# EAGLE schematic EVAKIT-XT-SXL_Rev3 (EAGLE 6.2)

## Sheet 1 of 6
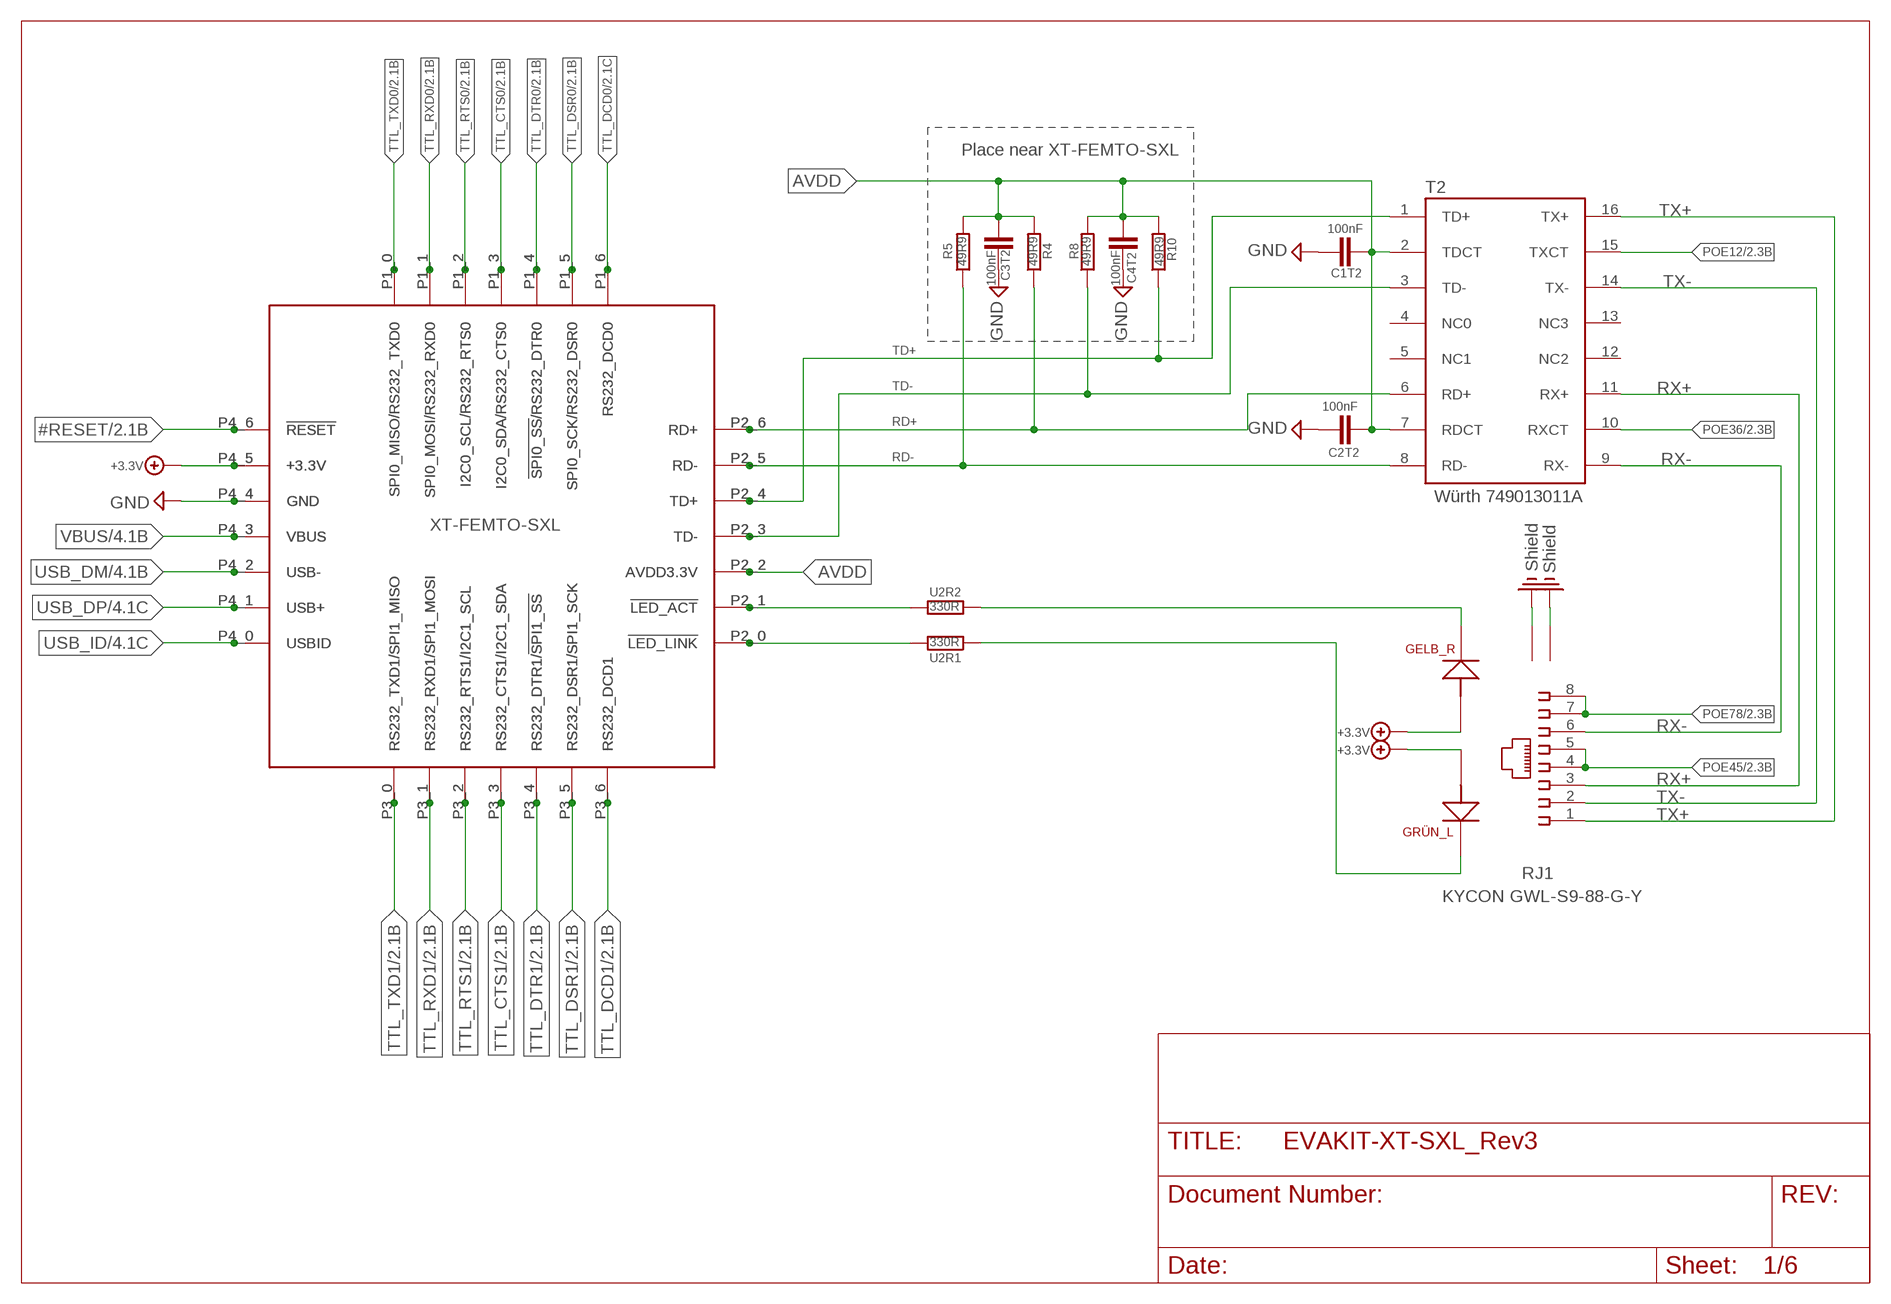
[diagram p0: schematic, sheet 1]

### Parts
C1T2  100nF  C0402AK  [AK0402]
C2T2  100nF  C0402AK  [AK0402]
C3T2  100nF  C0402AK  [AK0402]
C4T2  100nF  C0402AK  [AK0402]
M1  XT-FEMTO-SXL2  [XT-FEMTO-SXL-PAD]
R4  49R9  R0402AK  [AK0402]
R5  49R9  R0402AK  [AK0402]
R8  49R9  R0402AK  [AK0402]
R10  49R9  R0402AK  [AK0402]
RJ1  KYCON GWL-S9-88-G-Y  RJ45_ERNI_LED  [ORCAD_X_ERNI_RJ45_LED]
T2  Würth 749013011A  PULSE_H1102  [SOTRANSF]
U2R1  330R  R0402AK  [AK0402]
U2R2  330R  R0402AK  [AK0402]
XT-FEMTO-SXL  XT-FEMTO-SXL1  [XT-FEMTO-SXL-PIN]

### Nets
#RESET: M1.P4_6(!RESET) XT-FEMTO-SXL.P4_6(!RESET) ; also sheet 2,3,6
+3.3V: M1.P4_5(+3.3V) RJ1.A1 RJ1.A2 XT-FEMTO-SXL.P4_5(+3.3V) ; also sheet 2,3,4,5,6
AVDD: C1T2.1 C2T2.2 C3T2.1 C4T2.2 M1.P2_2(AVDD3.3V) R4.2 R5.2 R8.2 R10.2 T2.2(TDCT) T2.7(RDCT) XT-FEMTO-SXL.P2_2(AVDD3.3V)
GND: C1T2.2 C2T2.1 C3T2.2 C4T2.1 M1.P4_4(GND) XT-FEMTO-SXL.P4_4(GND) ; also sheet 2,3,4,5,6
N$1: M1.P2_1(!LED_ACT) U2R2.2 XT-FEMTO-SXL.P2_1(!LED_ACT)
N$2: RJ1.K2 U2R1.1
N$4: RJ1.K1 U2R2.1
N$6: M1.P2_0(!LED_LINK) U2R1.2 XT-FEMTO-SXL.P2_0(!LED_LINK)
PE: RJ1.9 RJ1.10 ; supply symbol labelled Shield ; also sheet 2,3,4,5
POE12: T2.15(TXCT) ; also sheet 2,3,6
POE36: T2.10(RXCT) ; also sheet 2,3,6
POE45: RJ1.4 RJ1.5 ; also sheet 2,3,6
POE78: RJ1.7 RJ1.8 ; also sheet 2,3,6
RD+: M1.P2_6(RD+) R4.1 T2.6(RD+) XT-FEMTO-SXL.P2_6(RD+)
RD-: M1.P2_5(RD-) R5.1 T2.8(RD-) XT-FEMTO-SXL.P2_5(RD-)
RX+: RJ1.3 T2.11(RX+)
RX-: RJ1.6 T2.9(RX-)
TD+: M1.P2_4(TD+) R10.1 T2.1(TD+) XT-FEMTO-SXL.P2_4(TD+)
TD-: M1.P2_3(TD-) R8.1 T2.3(TD-) XT-FEMTO-SXL.P2_3(TD-)
TTL_CTS0: M1.P1_3(I2C0_SDA/RS232_CTS0) XT-FEMTO-SXL.P1_3(I2C0_SDA/RS232_CTS0) ; also sheet 2,3,6
TTL_CTS1: M1.P3_3(RS232_CTS1/I2C1_SDA) XT-FEMTO-SXL.P3_3(RS232_CTS1/I2C1_SDA) ; also sheet 2,3,6
TTL_DCD0: M1.P1_6(RS232_DCD0) XT-FEMTO-SXL.P1_6(RS232_DCD0) ; also sheet 2,3,6
TTL_DCD1: M1.P3_6(RS232_DCD1) XT-FEMTO-SXL.P3_6(RS232_DCD1) ; also sheet 2,3,6
TTL_DSR0: M1.P1_5(SPI0_SCK/RS232_DSR0) XT-FEMTO-SXL.P1_5(SPI0_SCK/RS232_DSR0) ; also sheet 2,3,6
TTL_DSR1: M1.P3_5(RS232_DSR1/SPI1_SCK) XT-FEMTO-SXL.P3_5(RS232_DSR1/SPI1_SCK) ; also sheet 2,3,6
TTL_DTR0: M1.P1_4(!SPI0_SS!/RS232_DTR0) XT-FEMTO-SXL.P1_4(!SPI0_SS!/RS232_DTR0) ; also sheet 2,3,6
TTL_DTR1: M1.P3_4(RS232_DTR1/!SPI1_SS!) XT-FEMTO-SXL.P3_4(RS232_DTR1/!SPI1_SS!) ; also sheet 2,3,6
TTL_RTS0: M1.P1_2(I2C0_SCL/RS232_RTS0) XT-FEMTO-SXL.P1_2(I2C0_SCL/RS232_RTS0) ; also sheet 2,3,6
TTL_RTS1: M1.P3_2(RS232_RTS1/I2C1_SCL) XT-FEMTO-SXL.P3_2(RS232_RTS1/I2C1_SCL) ; also sheet 2,3,6
TTL_RXD0: M1.P1_1(SPI0_MOSI/RS232_RXD0) XT-FEMTO-SXL.P1_1(SPI0_MOSI/RS232_RXD0) ; also sheet 2,3,6
TTL_RXD1: M1.P3_1(RS232_RXD1/SPI1_MOSI) XT-FEMTO-SXL.P3_1(RS232_RXD1/SPI1_MOSI) ; also sheet 2,3,6
TTL_TXD0: M1.P1_0(SPI0_MISO/RS232_TXD0) XT-FEMTO-SXL.P1_0(SPI0_MISO/RS232_TXD0) ; also sheet 2,3,6
TTL_TXD1: M1.P3_0(RS232_TXD1/SPI1_MISO) XT-FEMTO-SXL.P3_0(RS232_TXD1/SPI1_MISO) ; also sheet 2,3,6
TX+: RJ1.1 T2.16(TX+)
TX-: RJ1.2 T2.14(TX-)
USB_DM: M1.P4_2(USB-) XT-FEMTO-SXL.P4_2(USB-) ; also sheet 4
USB_DP: M1.P4_1(USB+) XT-FEMTO-SXL.P4_1(USB+) ; also sheet 4
USB_ID: M1.P4_0(USBID) XT-FEMTO-SXL.P4_0(USBID) ; also sheet 4
VBUS: M1.P4_3(VBUS) XT-FEMTO-SXL.P4_3(VBUS) ; also sheet 4
Unconnected: T2.4(NC0) T2.5(NC1) T2.12(NC2) T2.13(NC3)

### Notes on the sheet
- Place near XT-FEMTO-SXL

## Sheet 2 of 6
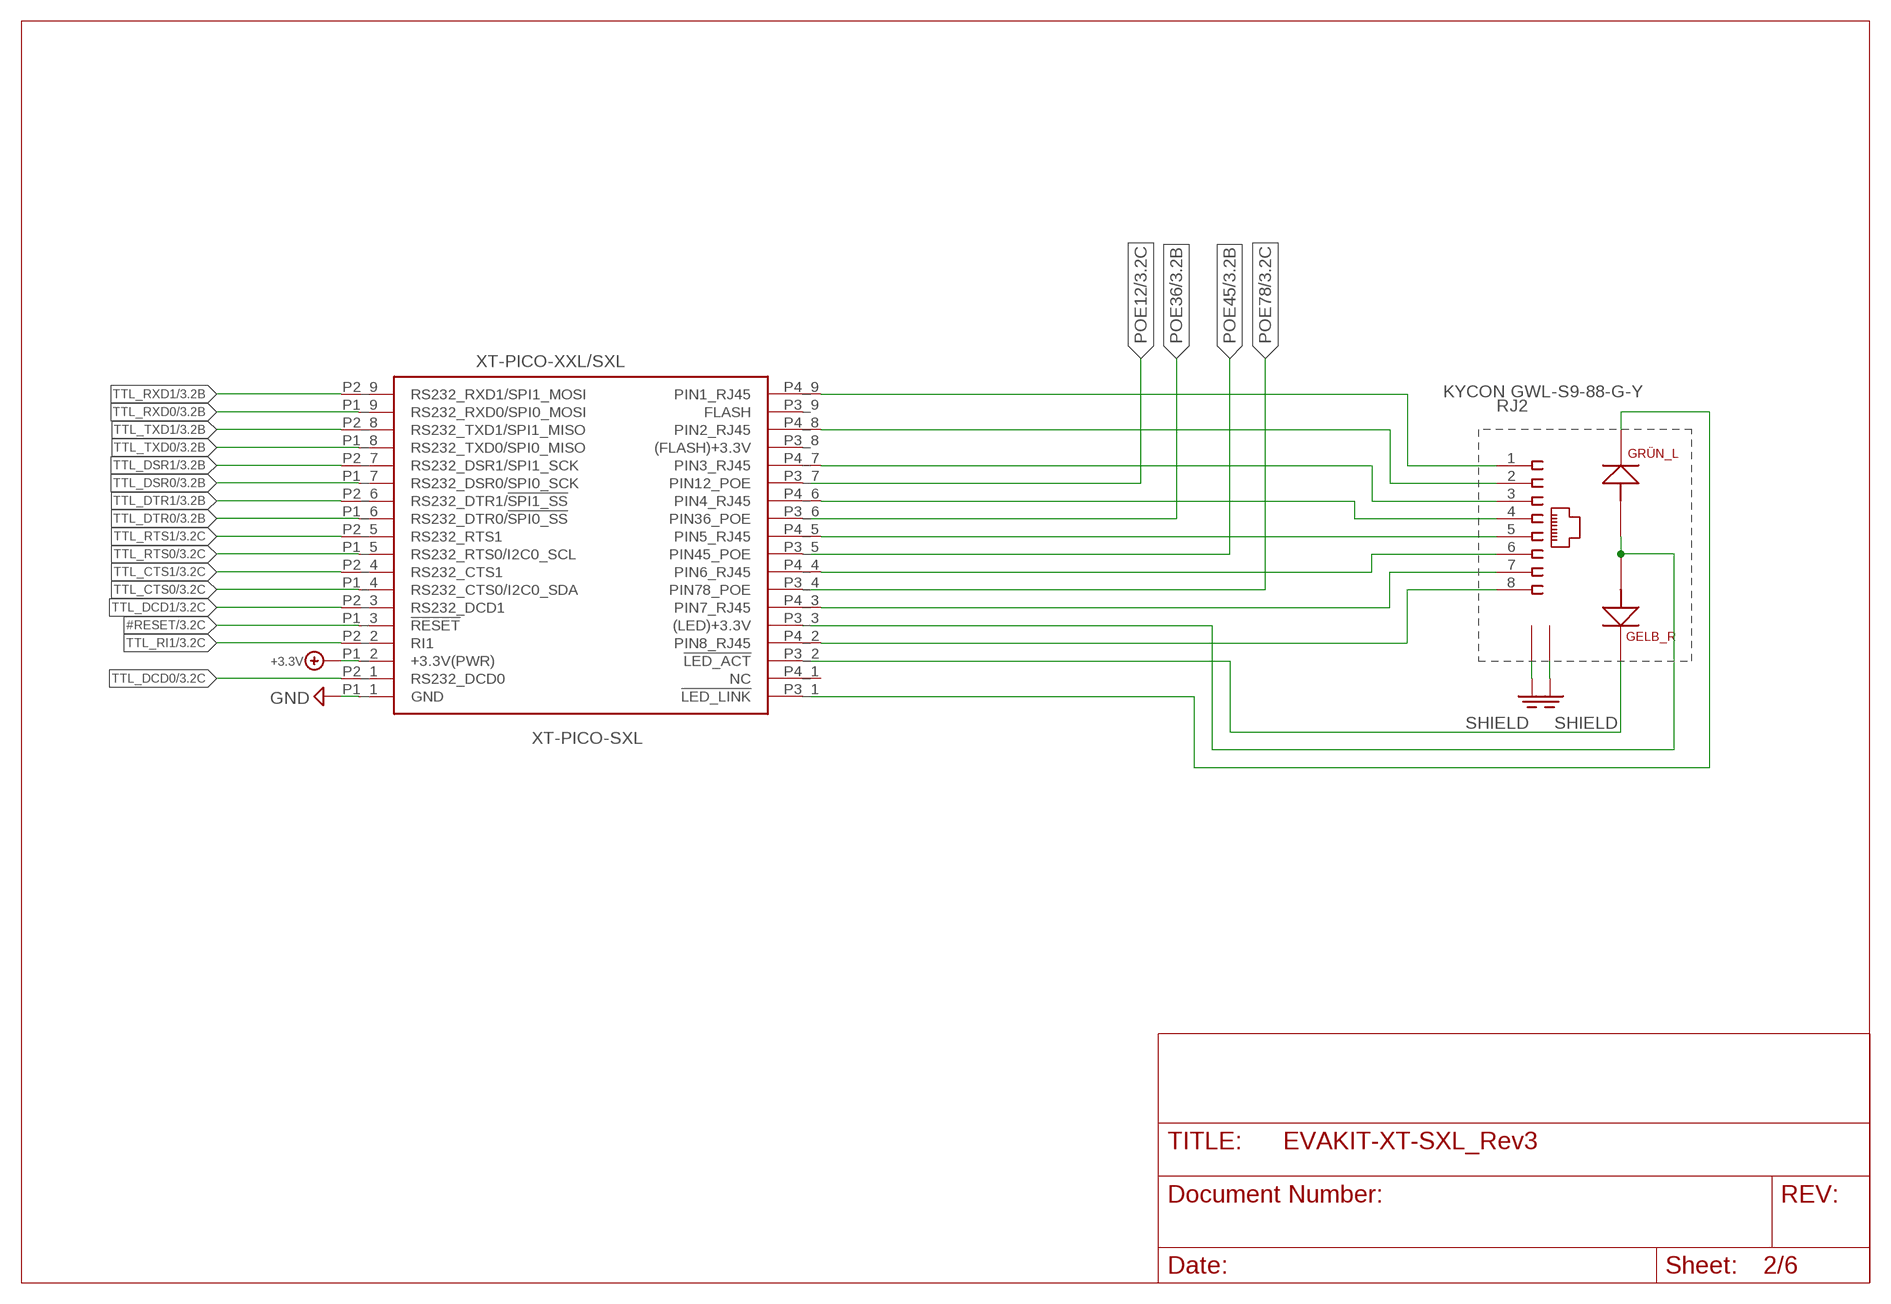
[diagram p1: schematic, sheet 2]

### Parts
RJ2  KYCON GWL-S9-88-G-Y  RJ45_ERNI_LED  [ORCAD_X_ERNI_RJ45_LED]
XT-PICO-SXL  XT-PICO-XXL/SXL  [XT-PICO-XXL/SXL]

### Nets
#RESET: XT-PICO-SXL.P1_3(!RESET) ; also sheet 1,3,6
+3.3V: XT-PICO-SXL.P1_2(+3.3V(PWR)) ; also sheet 1,3,4,5,6
GND: XT-PICO-SXL.P1_1(GND) ; also sheet 1,3,4,5,6
N$23: RJ2.1 XT-PICO-SXL.P4_9(PIN1_RJ45)
N$24: RJ2.2 XT-PICO-SXL.P4_8(PIN2_RJ45)
N$25: RJ2.3 XT-PICO-SXL.P4_7(PIN3_RJ45)
N$26: RJ2.6 XT-PICO-SXL.P4_4(PIN6_RJ45)
N$27: RJ2.K1 XT-PICO-SXL.P3_2(!LED_ACT)
N$28: RJ2.K2 XT-PICO-SXL.P3_1(!LED_LINK)
N$29: RJ2.A1 RJ2.A2 XT-PICO-SXL.P3_3((LED)+3.3V)
N$34: RJ2.4 XT-PICO-SXL.P4_6(PIN4_RJ45)
N$35: RJ2.5 XT-PICO-SXL.P4_5(PIN5_RJ45)
N$36: RJ2.7 XT-PICO-SXL.P4_3(PIN7_RJ45)
N$39: RJ2.8 XT-PICO-SXL.P4_2(PIN8_RJ45)
PE: RJ2.9 RJ2.10 ; supply symbol labelled SHIELD ; also sheet 1,3,4,5
POE12: XT-PICO-SXL.P3_7(PIN12_POE) ; also sheet 1,3,6
POE36: XT-PICO-SXL.P3_6(PIN36_POE) ; also sheet 1,3,6
POE45: XT-PICO-SXL.P3_5(PIN45_POE) ; also sheet 1,3,6
POE78: XT-PICO-SXL.P3_4(PIN78_POE) ; also sheet 1,3,6
TTL_CTS0: XT-PICO-SXL.P1_4(RS232_CTS0/I2C0_SDA) ; also sheet 1,3,6
TTL_CTS1: XT-PICO-SXL.P2_4(RS232_CTS1) ; also sheet 1,3,6
TTL_DCD0: XT-PICO-SXL.P2_1(RS232_DCD0) ; also sheet 1,3,6
TTL_DCD1: XT-PICO-SXL.P2_3(RS232_DCD1) ; also sheet 1,3,6
TTL_DSR0: XT-PICO-SXL.P1_7(RS232_DSR0/SPI0_SCK) ; also sheet 1,3,6
TTL_DSR1: XT-PICO-SXL.P2_7(RS232_DSR1/SPI1_SCK) ; also sheet 1,3,6
TTL_DTR0: XT-PICO-SXL.P1_6(RS232_DTR0/!SPI0_SS!) ; also sheet 1,3,6
TTL_DTR1: XT-PICO-SXL.P2_6(RS232_DTR1/!SPI1_SS!) ; also sheet 1,3,6
TTL_RI1: XT-PICO-SXL.P2_2(RI1) ; also sheet 3,6
TTL_RTS0: XT-PICO-SXL.P1_5(RS232_RTS0/I2C0_SCL) ; also sheet 1,3,6
TTL_RTS1: XT-PICO-SXL.P2_5(RS232_RTS1) ; also sheet 1,3,6
TTL_RXD0: XT-PICO-SXL.P1_9(RS232_RXD0/SPI0_MOSI) ; also sheet 1,3,6
TTL_RXD1: XT-PICO-SXL.P2_9(RS232_RXD1/SPI1_MOSI) ; also sheet 1,3,6
TTL_TXD0: XT-PICO-SXL.P1_8(RS232_TXD0/SPI0_MISO) ; also sheet 1,3,6
TTL_TXD1: XT-PICO-SXL.P2_8(RS232_TXD1/SPI1_MISO) ; also sheet 1,3,6
Unconnected: XT-PICO-SXL.P3_8((FLASH)+3.3V) XT-PICO-SXL.P3_9(FLASH) XT-PICO-SXL.P4_1(NC)

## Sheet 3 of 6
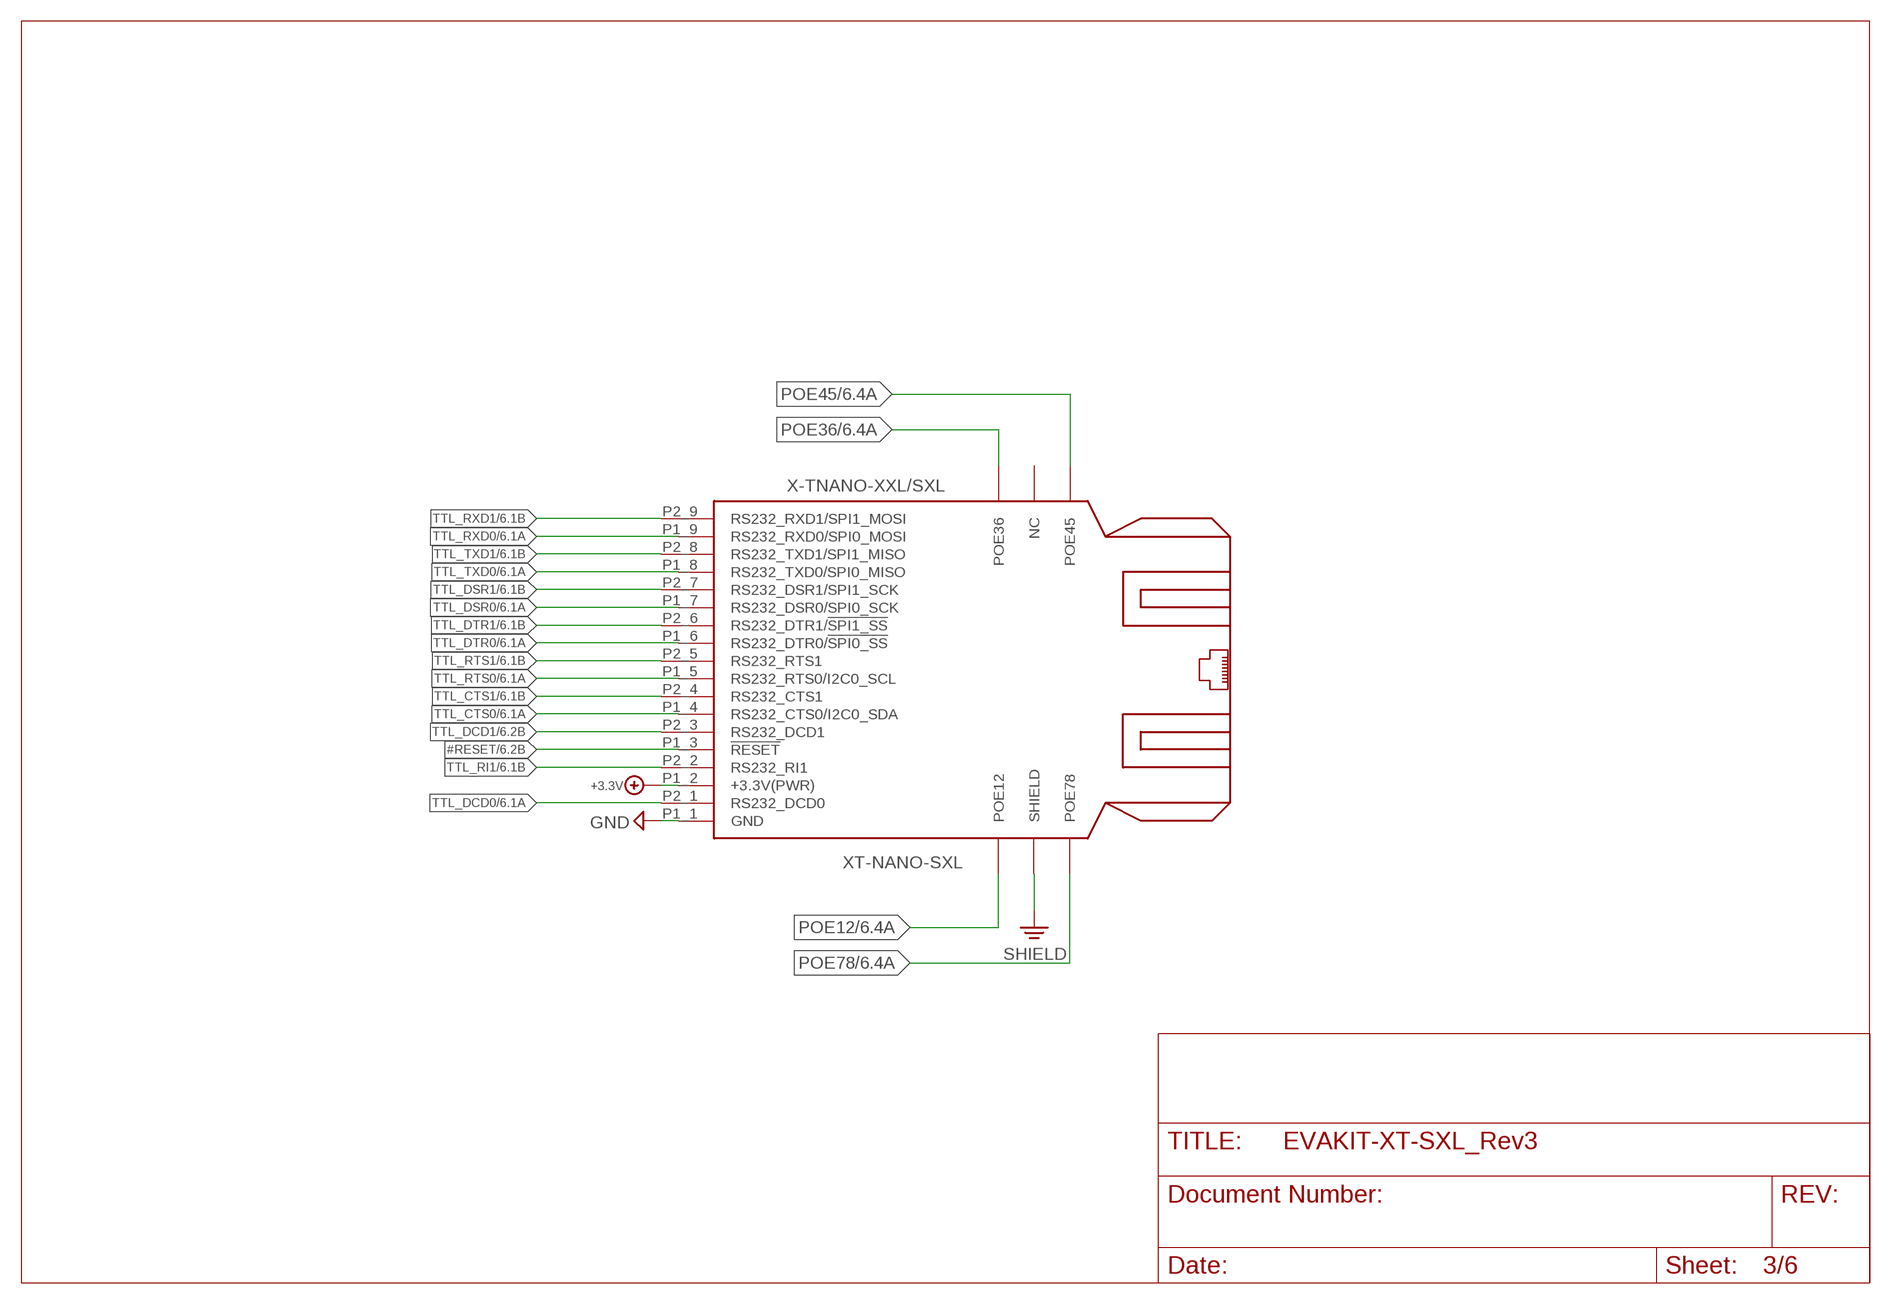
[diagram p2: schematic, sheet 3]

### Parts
XT-NANO-SXL  X-TNANO-XXL/SXL  [XT-NANO-XXL/SXL]

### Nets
#RESET: XT-NANO-SXL.P1_3(!RESET) ; also sheet 1,2,6
+3.3V: XT-NANO-SXL.P1_2(+3.3V(PWR)) ; also sheet 1,2,4,5,6
GND: XT-NANO-SXL.P1_1(GND) ; also sheet 1,2,4,5,6
PE: XT-NANO-SXL.SHIELD ; supply symbol labelled SHIELD ; also sheet 1,2,4,5
POE12: XT-NANO-SXL.POE12 ; also sheet 1,2,6
POE36: XT-NANO-SXL.POE36 ; also sheet 1,2,6
POE45: XT-NANO-SXL.POE45 ; also sheet 1,2,6
POE78: XT-NANO-SXL.POE78 ; also sheet 1,2,6
TTL_CTS0: XT-NANO-SXL.P1_4(RS232_CTS0/I2C0_SDA) ; also sheet 1,2,6
TTL_CTS1: XT-NANO-SXL.P2_4(RS232_CTS1) ; also sheet 1,2,6
TTL_DCD0: XT-NANO-SXL.P2_1(RS232_DCD0) ; also sheet 1,2,6
TTL_DCD1: XT-NANO-SXL.P2_3(RS232_DCD1) ; also sheet 1,2,6
TTL_DSR0: XT-NANO-SXL.P1_7(RS232_DSR0/SPI0_SCK) ; also sheet 1,2,6
TTL_DSR1: XT-NANO-SXL.P2_7(RS232_DSR1/SPI1_SCK) ; also sheet 1,2,6
TTL_DTR0: XT-NANO-SXL.P1_6(RS232_DTR0/!SPI0_SS!) ; also sheet 1,2,6
TTL_DTR1: XT-NANO-SXL.P2_6(RS232_DTR1/!SPI1_SS!) ; also sheet 1,2,6
TTL_RI1: XT-NANO-SXL.P2_2(RS232_RI1) ; also sheet 2,6
TTL_RTS0: XT-NANO-SXL.P1_5(RS232_RTS0/I2C0_SCL) ; also sheet 1,2,6
TTL_RTS1: XT-NANO-SXL.P2_5(RS232_RTS1) ; also sheet 1,2,6
TTL_RXD0: XT-NANO-SXL.P1_9(RS232_RXD0/SPI0_MOSI) ; also sheet 1,2,6
TTL_RXD1: XT-NANO-SXL.P2_9(RS232_RXD1/SPI1_MOSI) ; also sheet 1,2,6
TTL_TXD0: XT-NANO-SXL.P1_8(RS232_TXD0/SPI0_MISO) ; also sheet 1,2,6
TTL_TXD1: XT-NANO-SXL.P2_8(RS232_TXD1/SPI1_MISO) ; also sheet 1,2,6
Unconnected: XT-NANO-SXL.FLASH(NC)

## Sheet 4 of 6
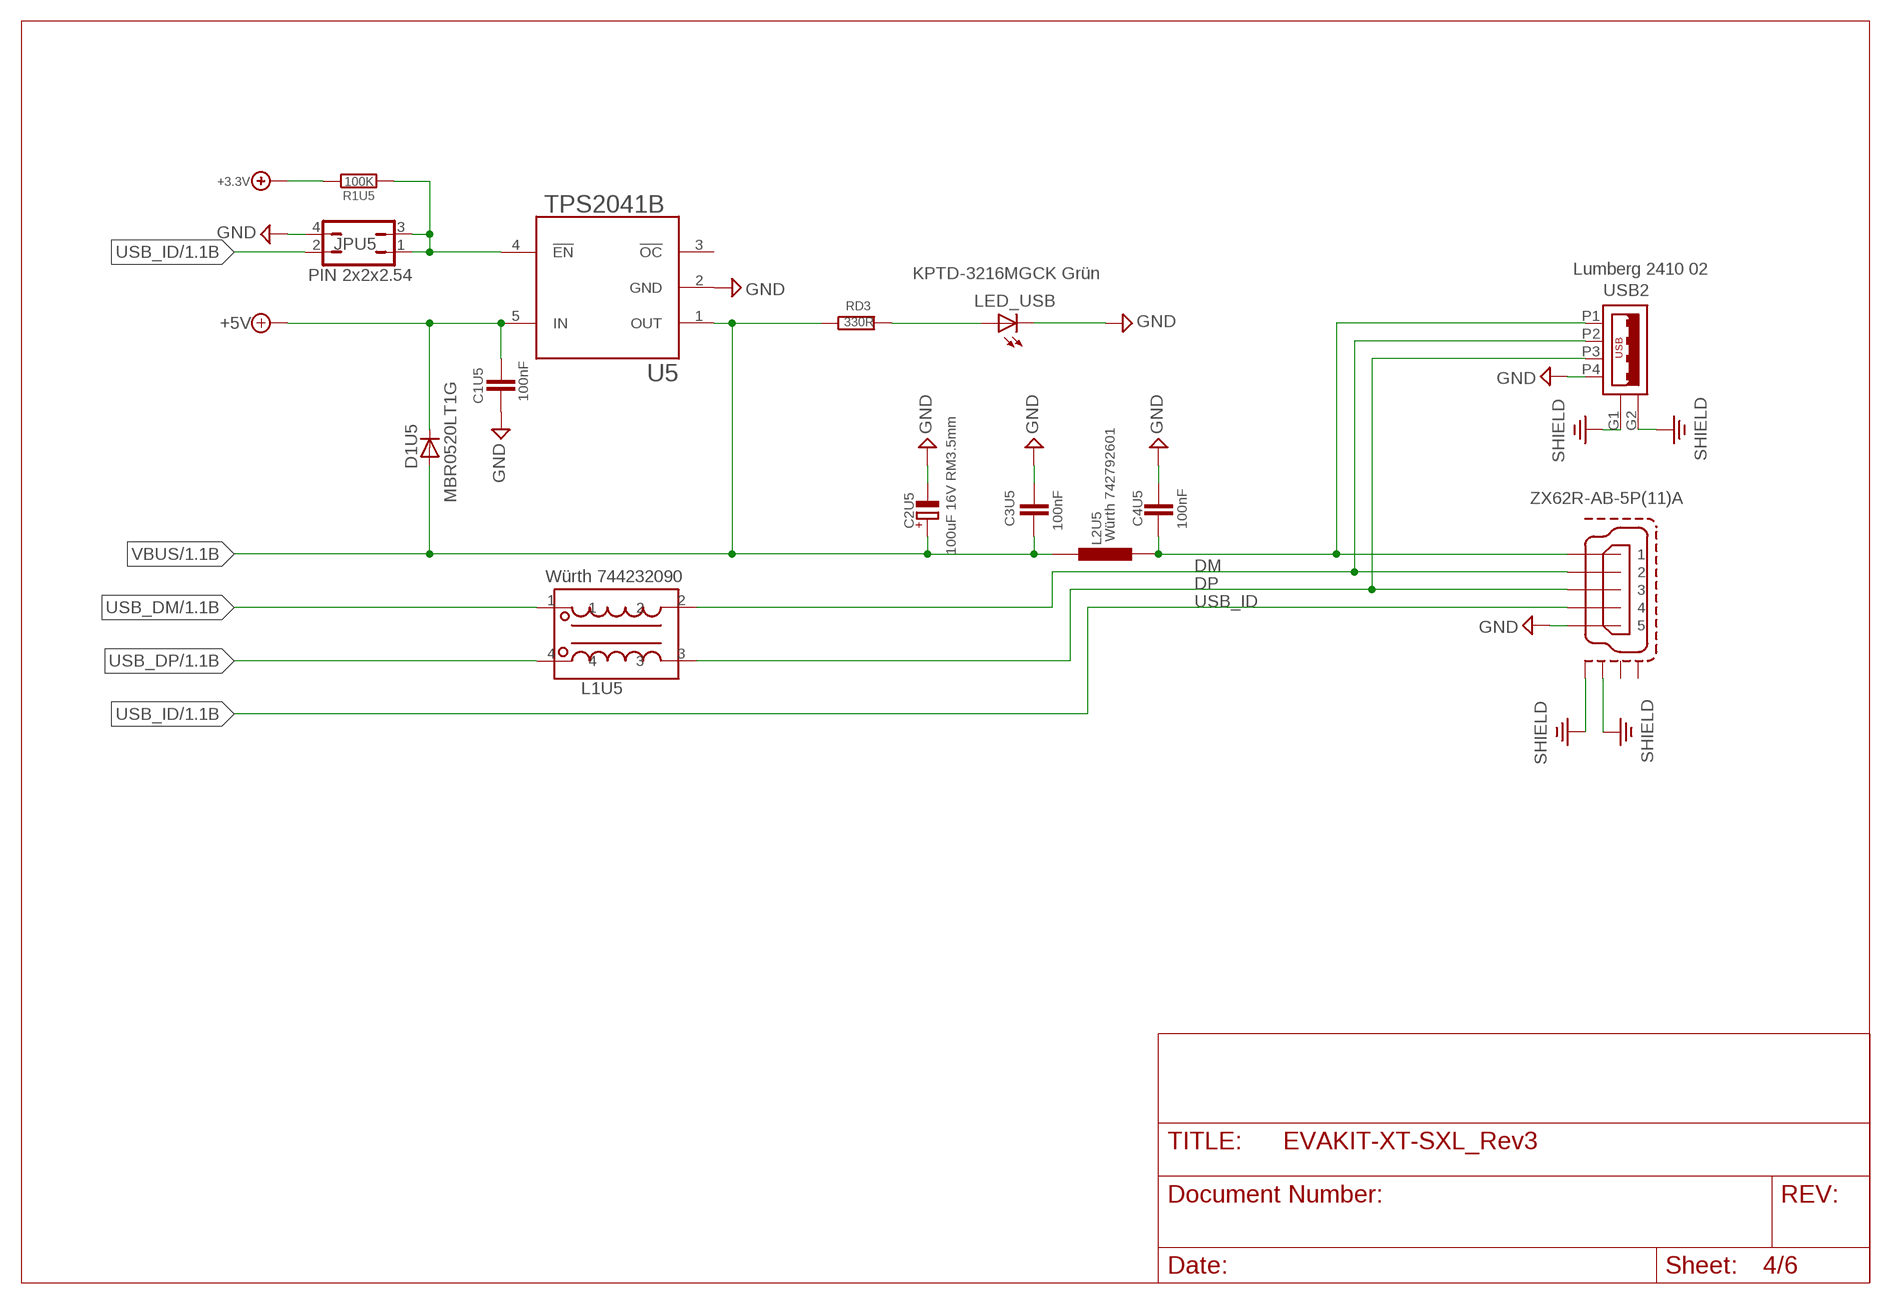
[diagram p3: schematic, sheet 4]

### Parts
C1U5  100nF  C0402AK  [AK0402]
C2U5  100uF 16V RM3.5mm  CPOL-EU153CLV-0605  [153CLV-0605]
C3U5  100nF  C0402AK  [AK0402]
C4U5  100nF  C0402AK  [AK0402]
D1U5  MBR0520LT1G  MBR0520LT  [SOD123]
JPU5  PIN 2x2x2.54  JP2Q  [JP2Q]
L1U5  Würth 744232090  WE-CNSW  [2L1206]
L2U5  Würth 742792601  CHIP-L-0603  [SMD-0603]
LED_USB  KPTD-3216MGCK Grün  LEDSMT1206  [1206]
R1U5  100K  R0402AK  [AK0402]
RD3  330R  R0402AK  [AK0402]
U5  TPS2041B  [SOT23-5]
USB1  ZX62R-AB-5P(11)A  [ZX62R-AB-5P(11)]
USB2  Lumberg 2410 02  USB_A_1  [USB_A_1]

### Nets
+3.3V: R1U5.1 ; also sheet 1,2,3,5,6
+5V: C1U5.1 D1U5.C U5.5(IN) ; also sheet 6
DM: L1U5.2 USB1.2 USB2.P2
DP: L1U5.3 USB1.3 USB2.P3
GND: C1U5.2 C2U5.- C3U5.1 C4U5.1 JPU5.4 LED_USB.C U5.2(GND) USB1.5 USB2.P4 ; also sheet 1,2,3,5,6
N$15: C4U5.2 L2U5.2 USB1.1 USB2.P1
N$16: JPU5.1 JPU5.3 R1U5.2 U5.4(!EN)
N$22: LED_USB.A RD3.2
PE: USB1.M1(S1) USB1.M2(S2) USB2.G1 USB2.G2 ; supply symbol labelled SHIELD ; also sheet 1,2,3,5
USB_DM: L1U5.1 ; also sheet 1
USB_DP: L1U5.4 ; also sheet 1
USB_ID: JPU5.2 USB1.4 ; also sheet 1
VBUS: C2U5.+ C3U5.2 D1U5.A L2U5.1 RD3.1 U5.1(OUT) ; also sheet 1
Unconnected: U5.3(!OC) USB1.M3(S3) USB1.M4(S4)

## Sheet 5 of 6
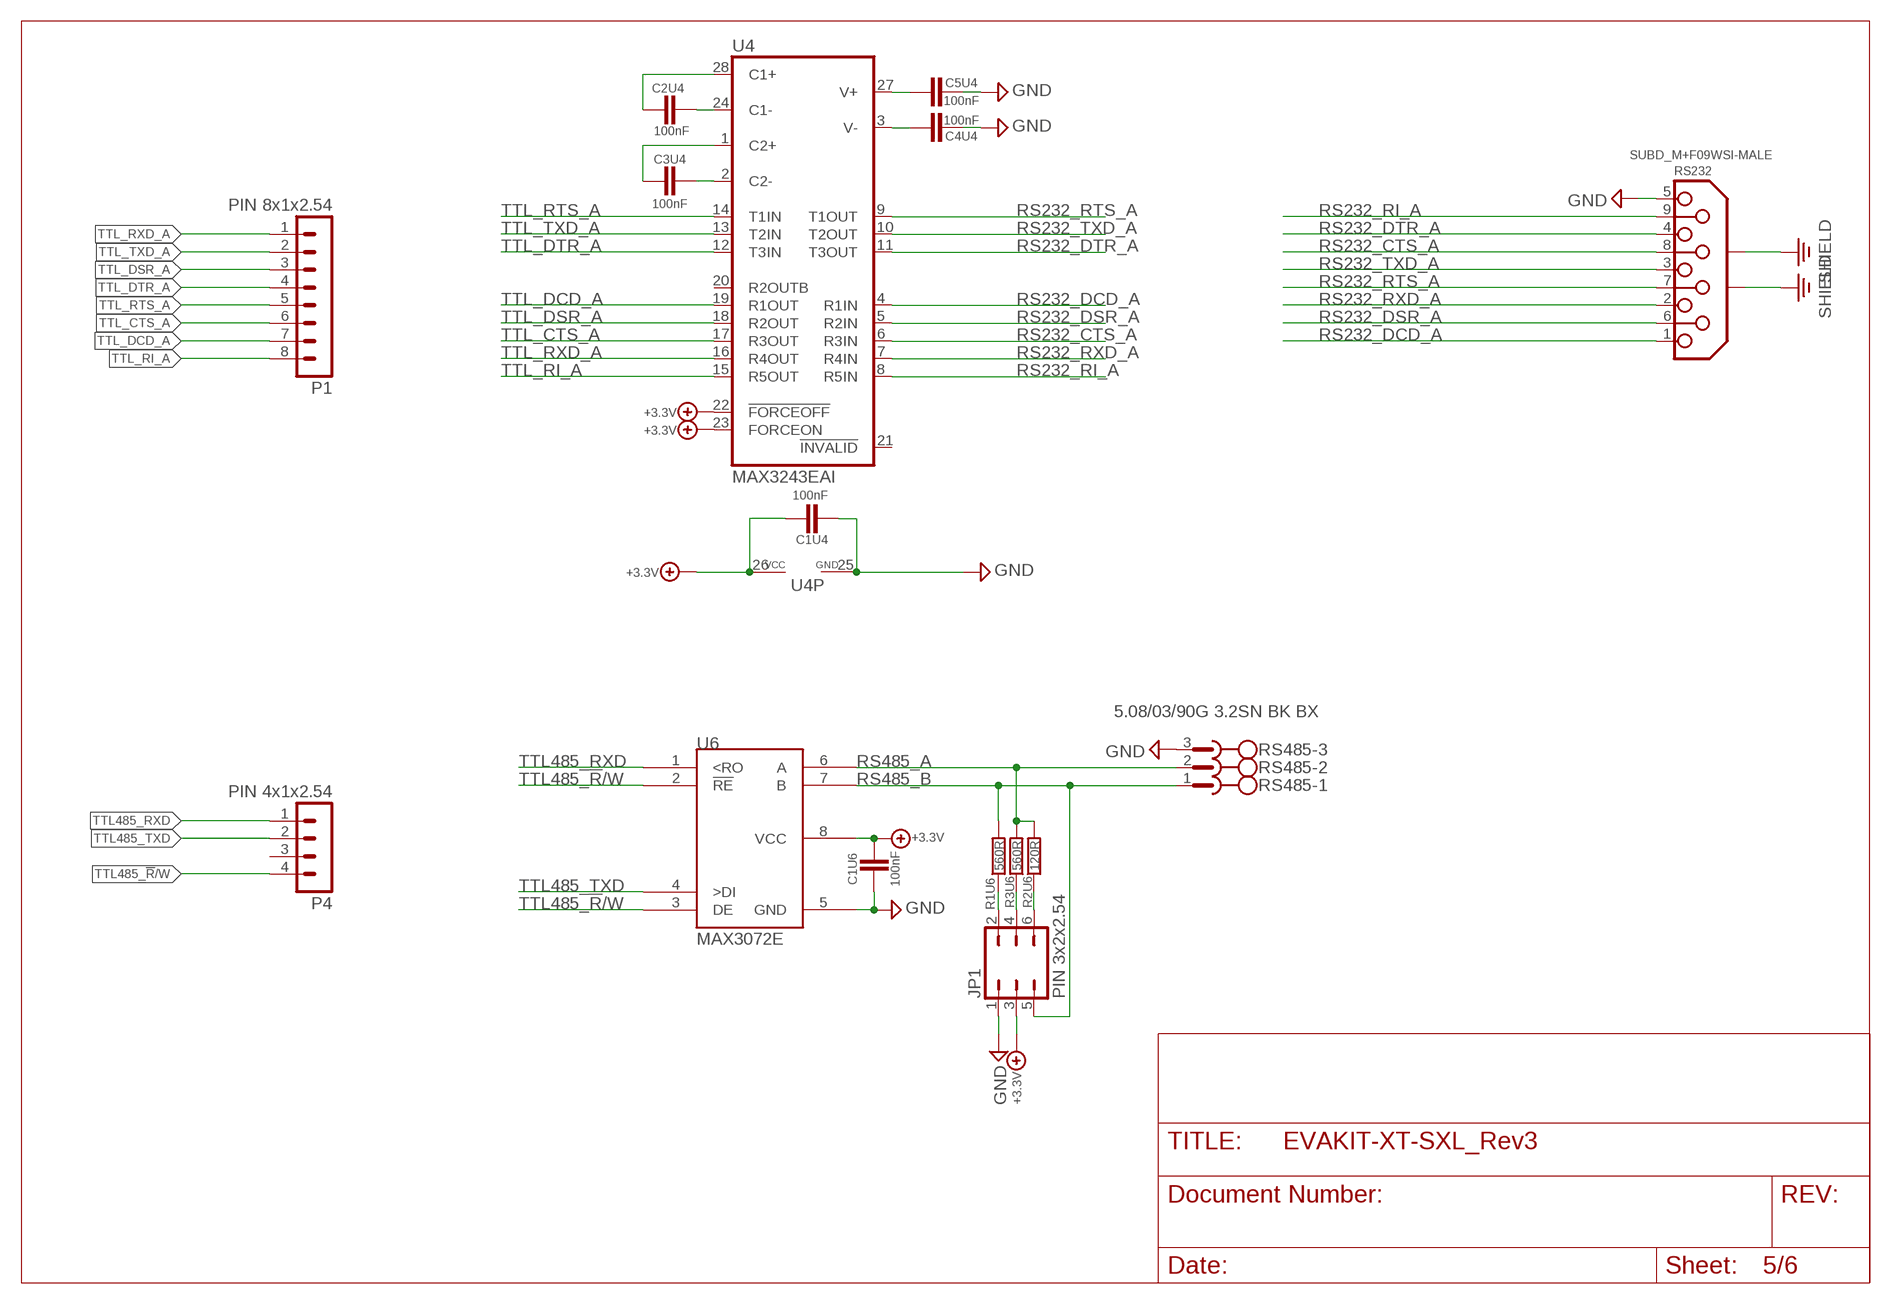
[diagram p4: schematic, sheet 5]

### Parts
C1U4  100nF  C0402AK  [AK0402]
C1U6  100nF  C0402AK  [AK0402]
C2U4  100nF  C0402AK  [AK0402]
C3U4  100nF  C0402AK  [AK0402]
C4U4  100nF  C0402AK  [AK0402]
C5U4  100nF  C0402AK  [AK0402]
JP1  PIN 3x2x2.54  JP3Q  [JP3Q]
P1  PIN 8x1x2.54  MA08-1  [MA08-1]
P4  PIN 4x1x2.54  MA04-1  [MA04-1]
R1U6  560R  R0402AK  [AK0402]
R2U6  120R  R0402AK  [AK0402]
R3U6  560R  R0402AK  [AK0402]
RS232  SUBD_M+F09WSI-MALE  [SUBD-M09HP-WSI]
RS485  5.08/03/90G 3.2SN BK BX  MSTBA3  [MSTBA3]
U4  MAX3243EAI  [SSOP28]
U6  MAX3072E  MAX3072E_SO8  [SO-8]

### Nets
+3.3V: C1U4.1 C1U6.2 JP1.3 U4.22(!FORCEOFF) U4.23(FORCEON) U4.26(VCC) U6.8(VCC) ; also sheet 1,2,3,4,6
GND: C1U4.2 C1U6.1 C4U4.2 C5U4.2 JP1.1 RS232.5 RS485.3 U4.25(GND) U6.5(GND) ; also sheet 1,2,3,4,6
N$3: C2U4.2 U4.28(C1+)
N$8: C3U4.2 U4.1(C2+)
N$10: C3U4.1 U4.2(C2-)
N$12: C2U4.1 U4.24(C1-)
N$13: C5U4.1 U4.27(V+)
N$14: C4U4.1 U4.3(V-)
N$17: JP1.2 R1U6.1
N$18: JP1.6 R2U6.1
N$19: JP1.4 R3U6.1
PE: RS232.G1 RS232.G2 ; supply symbol labelled SHIELD ; also sheet 1,2,3,4
RS232_CTS_A: RS232.8 U4.6(R3IN)
RS232_DCD_A: RS232.1 U4.4(R1IN)
RS232_DSR_A: RS232.6 U4.5(R2IN)
RS232_DTR_A: RS232.4 U4.11(T3OUT)
RS232_RI_A: RS232.9 U4.8(R5IN)
RS232_RTS_A: RS232.7 U4.9(T1OUT)
RS232_RXD_A: RS232.2 U4.7(R4IN)
RS232_TXD_A: RS232.3 U4.10(T2OUT)
RS485_A: R2U6.2 R3U6.2 RS485.2 U6.6(A)
RS485_B: JP1.5 R1U6.2 RS485.1 U6.7(B)
TTL485_!R!/W: P4.4 U6.2(!RE) U6.3(DE)
TTL485_RXD: P4.1 U6.1(<RO)
TTL485_TXD: P4.2 U6.4(>DI)
TTL_CTS_A: P1.6 U4.17(R3OUT)
TTL_DCD_A: P1.7 U4.19(R1OUT)
TTL_DSR_A: P1.3 U4.18(R2OUT)
TTL_DTR_A: P1.4 U4.12(T3IN)
TTL_RI_A: P1.8 U4.15(R5OUT)
TTL_RTS_A: P1.5 U4.14(T1IN)
TTL_RXD_A: P1.1 U4.16(R4OUT)
TTL_TXD_A: P1.2 U4.13(T2IN)
Unconnected: P4.3 U4.20(R2OUTB) U4.21(!INVALID)

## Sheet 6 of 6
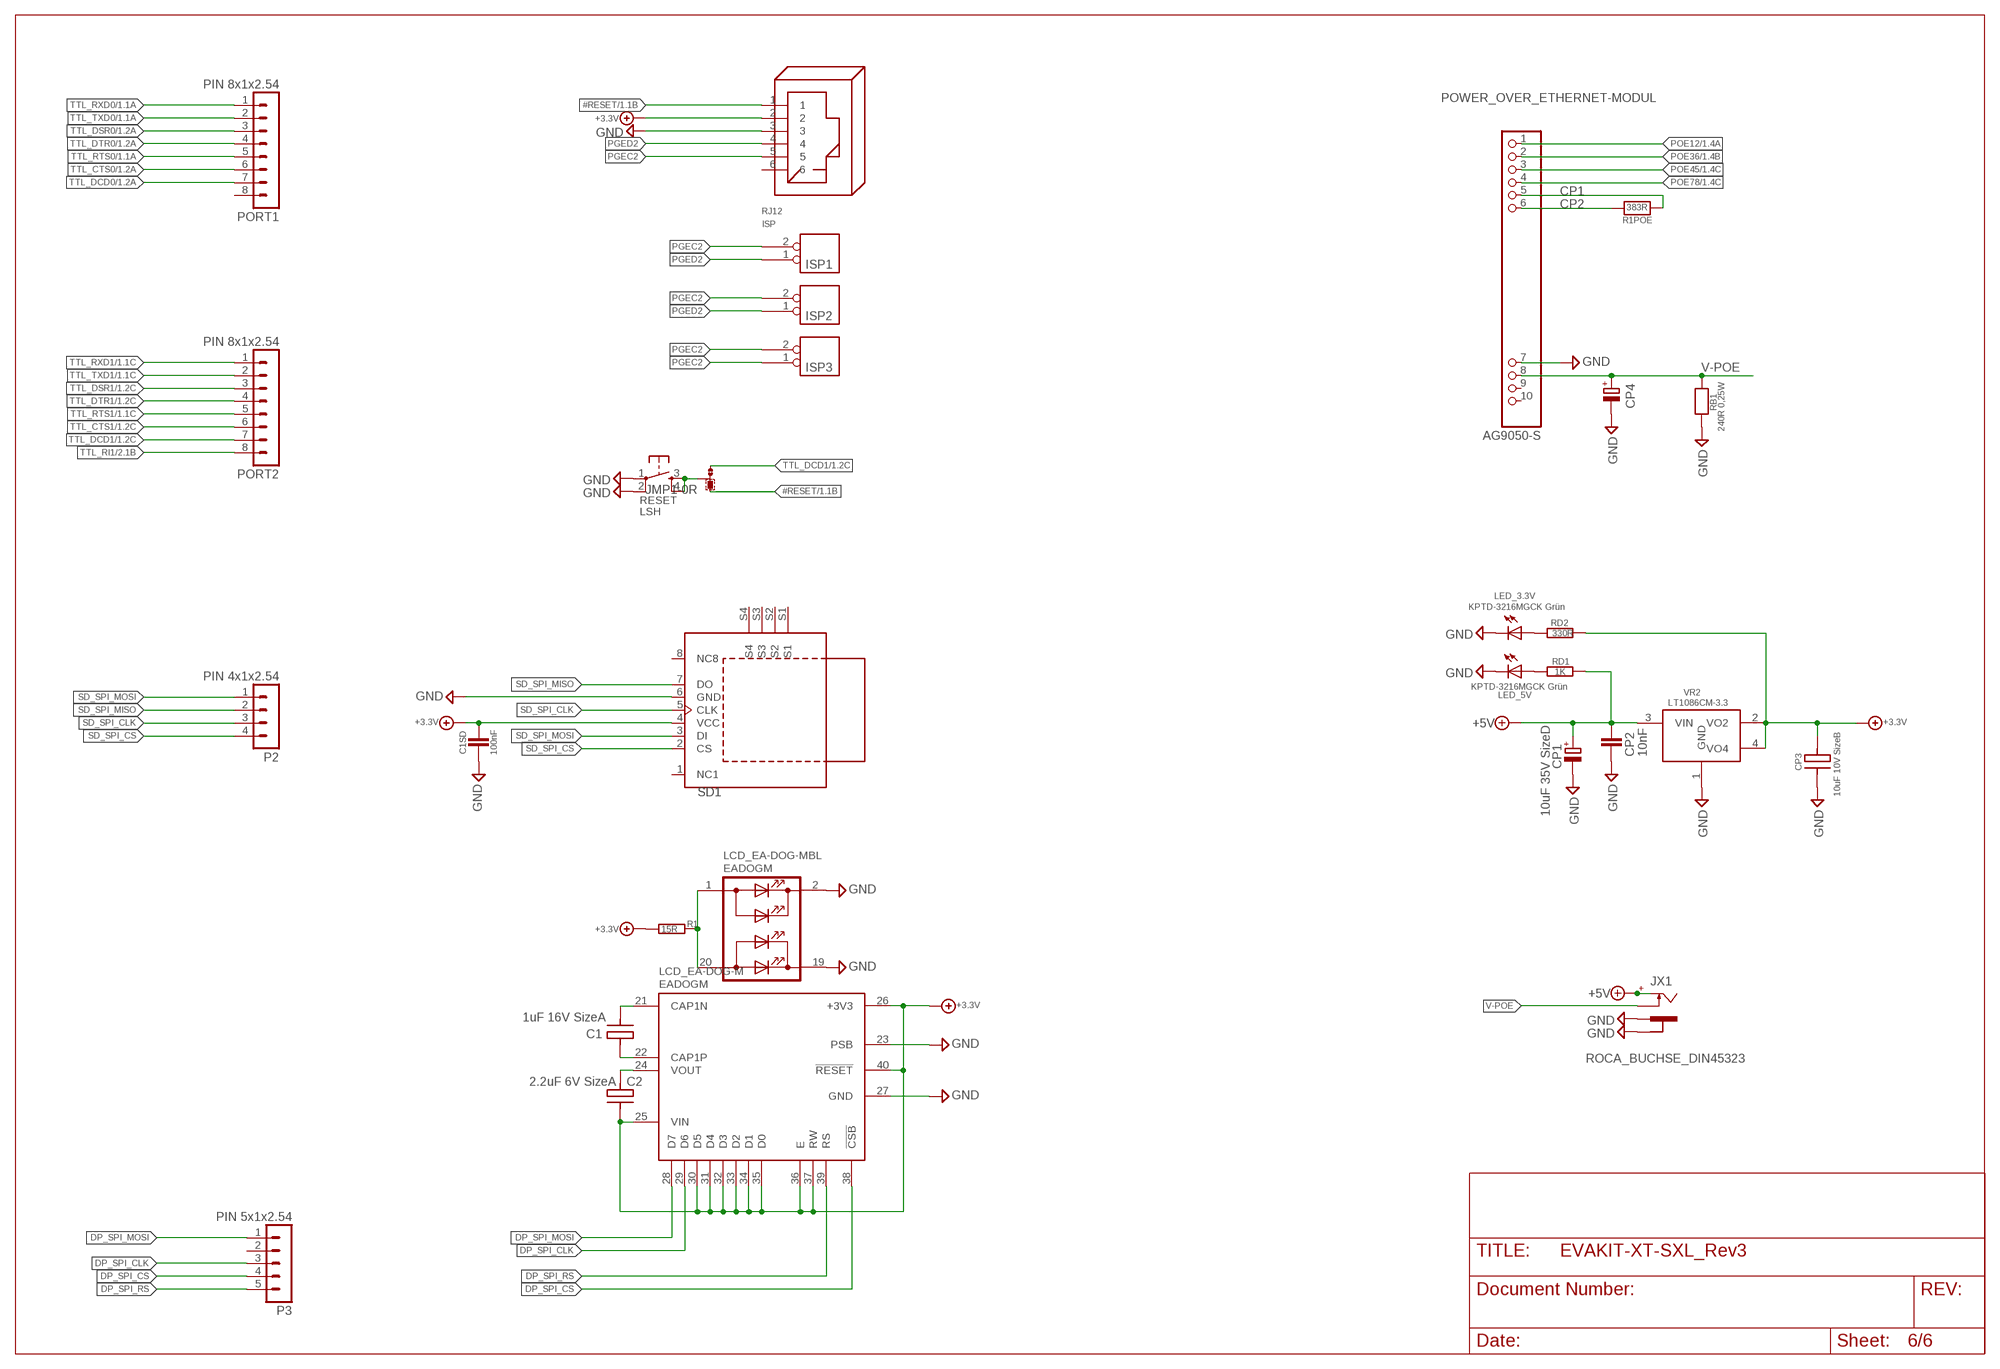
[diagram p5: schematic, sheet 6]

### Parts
C1  1uF 16V SizeA  C3216  [ORCAD_X_CT3216]
C1SD  100nF  C0402AK  [AK0402]
C2  2.2uF 6V SizeA  C3216  [ORCAD_X_CT3216]
CP1  10uF 35V SizeD  CPOL-EUD/7343-31R  [D/7343-31R]
CP2  10nF  C0402AK  [AK0402]
CP3  10uF 10V SizeB  C3528_B  [ORCAD_X_CT3528]
CP4  470uF 10V 3.5 x 8  CPOL-EU150CLZ-0810  [150CLZ-0810]
ISP  RJ12  [RJ12]
ISP1  JP2  [ROLF_SQW1X2]
ISP2  JP2  [ROLF_SQW1X2]
ISP3  JP2  [ROLF_SQW1X2]
JMP1  0R-JUMPA  [A0R-JMP]
JX1  ROCA_BUCHSE_DIN45323  ROKA  [ORCAD_X_ROKA1]
LCD_EA-DOG-M  EADOGM  [EADOGM]
LED_3.3V  KPTD-3216MGCK Grün  LEDSMT1206  [1206]
LED_5V  KPTD-3216MGCK Grün  LEDSMT1206  [1206]
P2  PIN 4x1x2.54  MA04-1  [MA04-1]
P3  PIN 5x1x2.54  MA05-1  [MA05-1]
PORT1  PIN 8x1x2.54  MA08-1  [MA08-1]
PORT2  PIN 8x1x2.54  MA08-1  [MA08-1]
POWER_OVER_ETHERNET-MODUL  AG9050-S  POE_AG9000  [POE_AG9000]
R1  15R  R0402AK  [AK0402]
R1POE  383R  CHIP-R-0603  [SMD-0603]
RB1  240R 0,25W  CHIP-R-0805  [SMD-0805]
RD1  1K  R0402AK  [AK0402]
RD2  330R  R0402AK  [AK0402]
RESET  LSH  [LSH]
SD1  MICROSD_SF-MICROSD  [MICROSD_MICROSD]
VR2  LT1086CM-3.3  LT1086_5.0  [DPAK_223]

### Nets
#RESET: ISP.1 JMP1.1 ; also sheet 1,2,3
+3.3V: C1SD.2 C2.2(C-) CP3.1(C+) ISP.2 LCD_EA-DOG-M.25(VIN) LCD_EA-DOG-M.26(+3V3) LCD_EA-DOG-M.30(D5) LCD_EA-DOG-M.31(D4) LCD_EA-DOG-M.32(D3) LCD_EA-DOG-M.33(D2) LCD_EA-DOG-M.34(D1) LCD_EA-DOG-M.35(D0) LCD_EA-DOG-M.36(E) LCD_EA-DOG-M.37(RW) LCD_EA-DOG-M.40(!RESET) R1.1 RD2.2 SD1.4(VCC) VR2.2(VO2) VR2.4(VO4) ; also sheet 1,2,3,4,5
+5V: CP1.+ CP2.2 JX1.1(+) RD1.2 VR2.3(VIN) ; also sheet 4
CP1: POWER_OVER_ETHERNET-MODUL.5(CP1) R1POE.1
CP2: POWER_OVER_ETHERNET-MODUL.6(CP2) R1POE.2
DP_SPI_CLK: LCD_EA-DOG-M.29(D6) P3.3
DP_SPI_CS: LCD_EA-DOG-M.38(!CSB) P3.4
DP_SPI_MOSI: LCD_EA-DOG-M.28(D7) P3.1
DP_SPI_RS: LCD_EA-DOG-M.39(RS) P3.5
GND: C1SD.1 CP1.- CP2.1 CP3.2(C-) CP4.- ISP.3 JX1.3(-1) JX1.4(-2) LCD_EA-DOG-M.2(C1) LCD_EA-DOG-M.19(C2) LCD_EA-DOG-M.23(PSB) LCD_EA-DOG-M.27(GND) LED_3.3V.C LED_5V.C POWER_OVER_ETHERNET-MODUL.7(GND) RB1.2 RESET.1(P) RESET.2(P1) SD1.6(GND) VR2.1(GND) ; also sheet 1,2,3,4,5
N$5: LCD_EA-DOG-M.1(A1) LCD_EA-DOG-M.20(A2) R1.2
N$7: C2.1(C+) LCD_EA-DOG-M.24(VOUT)
N$9: C1.2(C-) LCD_EA-DOG-M.21(CAP1N)
N$11: C1.1(C+) LCD_EA-DOG-M.22(CAP1P)
N$20: LED_5V.A RD1.1
N$21: LED_3.3V.A RD2.1
N$30: JMP1.2 RESET.3(S) RESET.4(S1)
PGEC2: ISP1.2 ISP2.2 ISP3.2 ISP.5
PGED2: ISP1.1 ISP2.1 ISP3.1 ISP.4
POE12: POWER_OVER_ETHERNET-MODUL.1(VA1) ; also sheet 1,2,3
POE36: POWER_OVER_ETHERNET-MODUL.2(VA2) ; also sheet 1,2,3
POE45: POWER_OVER_ETHERNET-MODUL.3(VB1) ; also sheet 1,2,3
POE78: POWER_OVER_ETHERNET-MODUL.4(VB2) ; also sheet 1,2,3
SD_SPI_CLK: P2.3 SD1.5(CLK)
SD_SPI_CS: P2.4 SD1.2(CS)
SD_SPI_MISO: P2.2 SD1.7(DO)
SD_SPI_MOSI: P2.1 SD1.3(DI)
TTL_CTS0: PORT1.6 ; also sheet 1,2,3
TTL_CTS1: PORT2.6 ; also sheet 1,2,3
TTL_DCD0: PORT1.7 ; also sheet 1,2,3
TTL_DCD1: JMP1.3 PORT2.7 ; also sheet 1,2,3
TTL_DSR0: PORT1.3 ; also sheet 1,2,3
TTL_DSR1: PORT2.3 ; also sheet 1,2,3
TTL_DTR0: PORT1.4 ; also sheet 1,2,3
TTL_DTR1: PORT2.4 ; also sheet 1,2,3
TTL_RI1: PORT2.8 ; also sheet 2,3
TTL_RTS0: PORT1.5 ; also sheet 1,2,3
TTL_RTS1: PORT2.5 ; also sheet 1,2,3
TTL_RXD0: PORT1.1 ; also sheet 1,2,3
TTL_RXD1: PORT2.1 ; also sheet 1,2,3
TTL_TXD0: PORT1.2 ; also sheet 1,2,3
TTL_TXD1: PORT2.2 ; also sheet 1,2,3
V-POE: CP4.+ JX1.2(K) POWER_OVER_ETHERNET-MODUL.8(VDC+) RB1.1
Unconnected: ISP.6 P3.2 PORT1.8 POWER_OVER_ETHERNET-MODUL.9(ADJ) POWER_OVER_ETHERNET-MODUL.10(IC) SD1.1(NC1) SD1.8(NC8) SD1.S1 SD1.S2 SD1.S3 SD1.S4

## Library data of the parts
C1 C2 = XTMACRO:C3216
C1SD C1T2 C1U4-C1U6 C2T2 C2U4 C3T2 C3U4 C3U5 C4T2 C4U4 C4U5 C5U4 CP2 = ak-nord:C0402AK
C2U5 CP4 = rcl:CPOL-EU: POLARIZED CAPACITOR, European symbol
CP1 = rlc_sprintec:CPOL-EU: POLARIZED CAPACITOR, European symbol
CP3 = XTMACRO_AS:C3528_B
D1U5 = diode:MBR0520LT: SCHOTTKY BARRIER RECTIFIER
ISP = con-rj:RJ12: RJ12, RJ14 and RJ25 RJ12, RJ14 and RJ25 jacks side mounted http://www.tycoelectronics.com
ISP1-ISP3 = XTMACRO_AS:JP2
JMP1 = jump-0r-smd:0R-JUMP: SMD 0R 0805 Jumper
JP1 = jumper:JP3Q: JUMPER
JPU5 = jumper:JP2Q: JUMPER
JX1 = XTMACRO_AS:ROKA
L1U5 = XTMACRO:WE-CNSW: SMD1206 WE-CNSW 100MHz 90Ohm ArtNr:744232090
L2U5 = XTMACRO:CHIP-L-?: Chip (and other) Inductors
LCD_EA-DOG-M = XTMACRO:EADOGM: THT EA LCD Display With LED Backlight
LED_3.3V LED_5V LED_USB = led:LED: LED
M1 XT-FEMTO-SXL = ak-devices:XT-FEMTO-SXL: AK-NORD XT-FEMTO-SXL
P1 PORT1 PORT2 = con-lstb:MA08-1: PIN HEADER; OC_FARNELL: unknown; OC_NEWARK: unknown
P2 P4 = con-lstb:MA04-1: PIN HEADER; OC_FARNELL: unknown; OC_NEWARK: unknown
P3 = con-lstb:MA05-1: PIN HEADER; OC_FARNELL: unknown; OC_NEWARK: unknown
POWER_OVER_ETHERNET-MODUL = XTMACRO:POE_AG9000: PIN HEADER
R1 R1U5 R1U6 R2U6 R3U6 R4 R5 R8 R10 RD1-RD3 U2R1 U2R2 = ak-nord:R0402AK
R1POE RB1 = mea-lib:CHIP-R-?: Chip resistors
RESET = calypso:LSH: SMD Schurter Momentary Switch
RJ1 RJ2 = XTMACRO:RJ45_ERNI_LED
RS232 = ak-nord:SUBD_M+F09WSI: SUB-D 9pol. Male/Female WSI
RS485 = con-phoenix-508:MSTBA3: PHOENIX
SD1 = sd:MICROSD_SF-MICROSD
T2 = XTMACRO_AS:PULSE_H1102
U4 = maxim:MAX3243*: RS-232 Transceivers with AutoShutdown 1µA Supply-Current, True +3V to +5.5V http://dbserv.maxim-ic.com/; MF: MAXIM; MPN: MAX3243EAI+; OC_FARNELL: unknown; OC_NEWARK: 67K4901
U5 = XTMACRO:TPS2041B: 5VOLT USB POWER SWITCH
U6 = XTMACRO_AS:MAX3072E_SO8
USB1 = ak-nord:ZX62R-AB-5P(11): Hirose Micro USB Connector ZX62R-AB-5P(11):Micro AB - Standard (Bottom mount), Shell SMT
USB2 = XTMACRO:USB_A_1: USB_A_1
VR2 = XTMACRO_AS:LT1086_5.0
XT-NANO-SXL = ak-devices:X-TNANO-XXL/SXL: AK-NORD XT-NANO-XXL/SXL
XT-PICO-SXL = ak-devices:XT-PICO-XXL/SXL: AK-NORD XT-PICO-XXL/SXL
